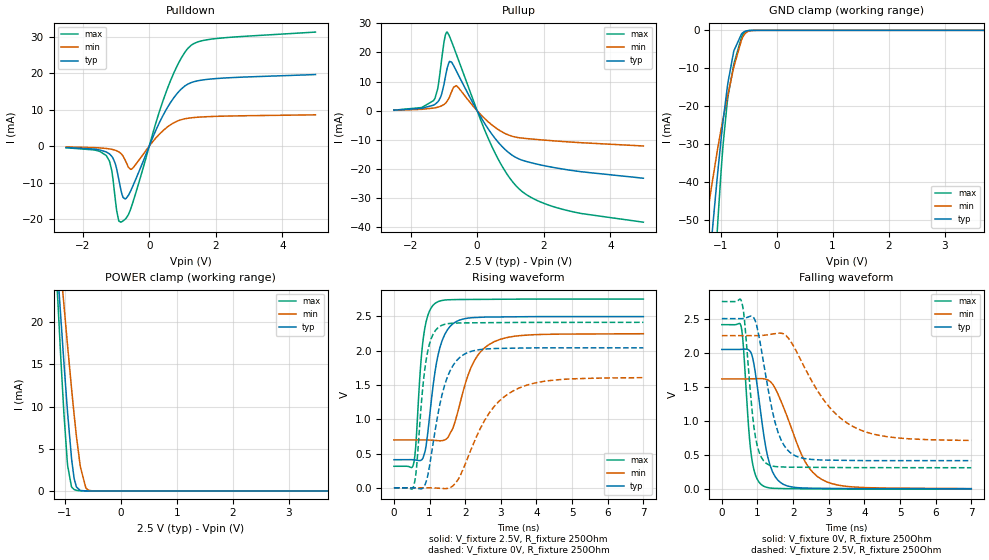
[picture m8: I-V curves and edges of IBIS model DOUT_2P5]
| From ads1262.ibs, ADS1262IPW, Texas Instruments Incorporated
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|   Model DOUT_2P5
[Model]   DOUT_2P5
Model_type   3-state
Polarity   Non-Inverting
Enable   Active-Low
Vmeas = 1.25
Vref = 2.5
Cref = 15pF
Rref = 250
|   typ   min   max
|   (slow PVT)   (nom PVT)   (fast PVT)
C_comp   0.298p   0.274p   0.333p
|C_comp (ON state)   0.298p   0.282p   0.346p
|C_comp (OFF state)   0.298p   0.274p   0.333p
| Where   nom PVT is  Nominal Process, 2.5V, 27C
|   Fast PVT is Strong Process, 2.25V, -40C
|   Slow PVT is Weak Process, 2.75V, 125C
[Voltage Range]   2.5   2.25   2.75
[Temperature Range]   27   125   -40
[Pullup Reference]   2.5   2.25   2.75
[Pulldown Reference]   -0   -0   -0
[Power Clamp Reference]   2.5   2.25   2.75
[GND Clamp Reference]   -0   -0   -0
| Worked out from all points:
|   slope of the pulldown table from 0 to 0.375 V, typ, clamps not added: 48.5 ohm
|   slope of the pullup table from 0 to 0.375 V, typ, clamps not added: 53.9 ohm
|   GND clamp passes 1 mA (typ) near -0.63 V on its own axis
|   POWER clamp passes 1 mA (typ) near -0.81 V on its own axis
|   falling waveform, V_fixture 0V, R_fixture 250Ohm: 20-80 % time 360ps typ, 768ps min, 205ps max; typ from 2.05 V to 0.008 V
|   rising waveform, V_fixture 2.5V, R_fixture 250Ohm: 20-80 % time 356ps typ, 621ps min, 211ps max; typ from 0.41 V to 2.49 V
|   rising waveform, V_fixture 0V, R_fixture 250Ohm: 20-80 % time 487ps typ, 1.02ns min, 263ps max; typ from 0 V to 2.04 V
|   falling waveform, V_fixture 2.5V, R_fixture 250Ohm: 20-80 % time 480ps typ, 1.21ns min, 261ps max; typ from 2.5 V to 0.419 V
[Pulldown]
|   Voltage   I(typ)   I(min)   I(max)
-2.5V     -374.4uA   -218.1uA   -432.2uA
-1.285V   -1.63mA    -652uA     -2.673mA
-1.127V   -2.768mA   -874uA     -6.634mA
-1.022V   -4.749mA   -1.125mA   -14.39mA
-917.5mV  -8.99mA    -1.557mA   -20.47mA
-850mV    -12.08mA   -2.03mA    -20.91mA
-722.5mV  -14.53mA   -3.836mA   -20.1mA
-542.5mV  -12.01mA   -6.358mA   -16.88mA
432.5mV   8.759mA    4.41mA     12.97mA
1.16V     17.05mA    7.666mA    26.88mA
1.895V    18.49mA    8.154mA    29.45mA
4.992V    19.68mA    8.607mA    31.35mA
[GND Clamp]
|   Voltage   I(typ)   I(min)   I(max)
-2.5V     -315.4mA   -202.2mA   -454.1mA
-1.345V   -87.13mA   -59.77mA   -127.8mA
-1.232V   -67.2mA    -48.19mA   -97.37mA
-1.157V   -54.48mA   -40.87mA   -77.6mA
-1.052V   -37.74mA   -31.27mA   -51.28mA
-955mV    -23.85mA   -23.3mA    -30.13mA
-865mV    -13.51mA   -16.67mA   -17.24mA
-760mV    -5.327mA   -9.473mA   -8.699mA
-625mV    -936.8uA   -2.504mA   -1.773mA
-572.5mV  -339uA     -1.047mA   -600.2uA
-332.5mV  -440.2nA   -5.503uA   -193.2nA
4.992V    0A         0A         0A
[Pullup]
|   Voltage   I(typ)   I(min)   I(max)
-2.5V     188.3uA    145.7uA    189.9uA
-1.308V   1.929mA    918.9uA    3.493mA
-1.188V   2.984mA    1.204mA    7.413mA
-1.09V    4.925mA    1.57mA     15.42mA
-992.5mV  9.311mA    2.188mA    23.78mA
-902.5mV  14.48mA    3.246mA    26.99mA
-827.5mV  16.94mA    4.824mA    25.47mA
-625mV    13.67mA    8.603mA    19.41mA
425mV     -7.769mA   -4.705mA   -11.84mA
1.265V    -16.6mA    -9.271mA   -26.89mA
2.525V    -19.93mA   -10.52mA   -33.72mA
4.992V    -23.17mA   -12.1mA    -38.27mA
[POWER Clamp]
|   Voltage   I(typ)   I(min)   I(max)
-2.5V     123.4mA    107.7mA    141.1mA
-1.465V   59.3mA     55.56mA    66.39mA
-1.067V   20.32mA    26.07mA    15.42mA
-1.015V   15.27mA    22.11mA    9.247mA
-947.5mV  9.154mA    17.1mA     2.987mA
-880mV    3.988mA    12.28mA    510.4uA
-827.5mV  1.346mA    8.743mA    154.9uA
-790mV    460.3uA    6.415mA    66.85uA
-722.5mV  52.29uA    2.915mA    11.74uA
-625mV    2.68uA     402.6uA    593.9nA
-550mV    280.8nA    52.81uA    22.11nA
4.992V    0A         0A         0A
[Ramp]
R_load = 250
|   typ   min   max
dV/dt_r   1.2507/3.55822e-10   0.92814/6.20741e-10   1.46138/2.11309e-10
dV/dt_f   1.22436/3.60122e-10   0.964363/7.68394e-10   1.44625/2.04746e-10
[Falling Waveform]
V_fixture = 0V
V_fixture_min = 0V
V_fixture_max = 0V
R_fixture = 250Ohm
C_fixture = 0F
|   Time   V(typ)   V(min)   V(max)
0s        2.048V     1.616V     2.411V
543.1ps   2.049V     1.616V     2.381V
829.2ps   1.986V     1.618V     487.3mV
946.7ps   1.682V     1.619V     203.4mV
1.164ns   842.5mV    1.619V     46.99mV
1.349ns   356.6mV    1.581V     18.45mV
1.58ns    128.8mV    1.389V     11.6mV
2.343ns   17.66mV    398mV      6.084mV
2.821ns   13.21mV    138.2mV    4.244mV
7ns       7.538mV    9.033mV    890.6uV
[Rising Waveform]
V_fixture = 2.5V
V_fixture_min = 2.25V
V_fixture_max = 2.75V
R_fixture = 250Ohm
C_fixture = 0F
|   Time   V(typ)   V(min)   V(max)
0s        409.6mV    697.9mV    313.9mV
543.1ps   409mV      697.7mV    333.8mV
611ps     405.3mV    697.7mV    597.1mV
829.2ps   455.8mV    697.7mV    2.198V
1.164ns   1.723V     690.4mV    2.691V
1.349ns   2.139V     687.2mV    2.729V
1.66ns    2.391V     875.7mV    2.741V
2.162ns   2.476V     1.75V      2.744V
2.821ns   2.488V     2.13V      2.746V
7ns       2.494V     2.245V     2.75V
[Rising Waveform]
V_fixture = 0V
V_fixture_min = 0V
V_fixture_max = 0V
R_fixture = 250Ohm
C_fixture = 0F
|   Time   V(typ)   V(min)   V(max)
0s        1.102nV    2.723nV    874.2pV
562ps     -193.5uV   92.02uV    38.62mV
635.5ps   -4.992mV   104.1uV    298.2mV
902.3ps   86.54mV    147.7uV    1.857V
1.242ns   1.09V      -5.347mV   2.336V
1.503ns   1.617V     -8.796mV   2.39V
1.82ns    1.886V     139.1mV    2.401V
2.681ns   2.025V     1.095V     2.406V
3.381ns   2.034V     1.421V     2.409V
7ns       2.039V     1.605V     2.411V
[Falling Waveform]
|Gnd
V_fixture = 2.5V
V_fixture_min = 2.25V
V_fixture_max = 2.75V
R_fixture = 250Ohm
C_fixture = 0F
|   Time   V(typ)   V(min)   V(max)
0s        2.5V       2.25V      2.75V
562ps     2.499V     2.25V      2.735V
902.3ps   2.507V     2.25V      904.7mV
1.045ns   2.232V     2.25V      544.2mV
1.242ns   1.635V     2.26V      380.3mV
1.66ns    725.6mV    2.286V     327.6mV
2.14ns    473.3mV    1.971V     322.2mV
2.961ns   426.6mV    1.239V     319.1mV
3.801ns   420.4mV    887.4mV    316.2mV
7ns       418.9mV    714.4mV    314.8mV
